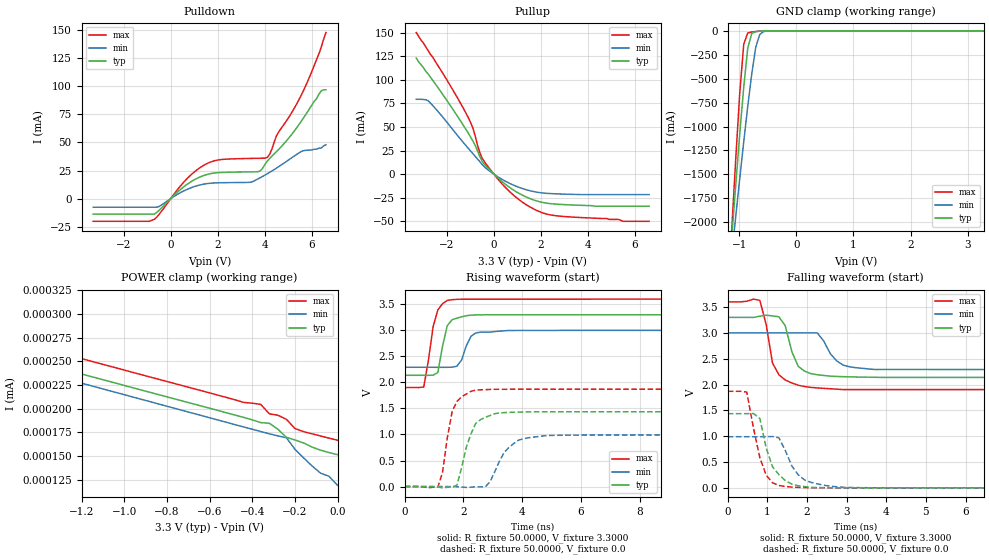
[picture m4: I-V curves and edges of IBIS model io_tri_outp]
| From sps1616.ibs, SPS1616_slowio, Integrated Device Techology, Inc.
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|   Model io_tri_outp
[Model]  io_tri_outp
Model_type 3-state
Polarity   Non-Inverting
Enable   Active-Low
Vmeas =  1.6500V
Cref =   50.0000pF
Rref =   1.0000M
Vref =   0.0V
C_comp   2.4707pF   2.4446pF   2.5092pF
[Temperature Range]   25.0000   0.1250k   -40.0000
[Voltage Range]   3.3000V   3.0000V   3.6000V
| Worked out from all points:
|   slope of the pulldown table from 0 to 0.495 V, typ, clamps not added: 51.9 ohm
|   slope of the pullup table from 0 to 0.495 V, typ, clamps not added: 45.6 ohm
|   GND clamp passes 1 mA (typ) near -0.54 V on its own axis
|   POWER clamp passes 1 mA (typ) near -2.49 V on its own axis
|   rising waveform, R_fixture 50.0000, V_fixture 3.3000: 20-80 % time 254ps typ, 295ps min, 311ps max; typ from 2.14 V to 3.3 V
|   rising waveform, R_fixture 50.0000, V_fixture 0.0: 20-80 % time 465ps typ, 642ps min, 346ps max; typ from 0 V to 1.44 V
|   falling waveform, R_fixture 50.0000, V_fixture 3.3000: 20-80 % time 295ps typ, 393ps min, 317ps max; typ from 3.3 V to 2.14 V
|   falling waveform, R_fixture 50.0000, V_fixture 0.0: 20-80 % time 393ps typ, 459ps min, 342ps max; typ from 1.44 V to 0 V
[Pulldown]
|Voltage   I(typ)   I(min)   I(max)
-3.3V     -13.86mA   -7.71mA    -20.27mA
-900mV    -13.86mA   -7.71mA    -20.27mA
-600mV    -12.36mA   -7.71mA    -16.59mA
700mV     12.78mA    8.245mA    17.92mA
1.5V      21.21mA    13.2mA     30.77mA
2.1V      23.2mA     14.09mA    34.69mA
3.7V      23.92mA    17.44mA    35.89mA
4.1V      33.25mA    22.07mA    36.63mA
4.5V      41.93mA    27.2mA     56.15mA
5.7V      73.6mA     42.86mA    98.81mA
6.4V      96mA       45mA       135mA
6.6V      97mA       48mA       148mA
[Pullup]
|Voltage   I(typ)   I(min)   I(max)
-3.3V     123mA      79.3mA     150mA
-2.8V     106.3mA    77.79mA    131mA
-1.2V     47.86mA    30.59mA    65.19mA
-900mV    35.42mA    21.89mA    49.37mA
-600mV    18.69mA    13.25mA    22.89mA
-500mV    13.73mA    10.33mA    16.95mA
300mV     -6.88mA    -4.819mA   -8.986mA
1V        -19.4mA    -13.37mA   -25.69mA
1.7V      -27.44mA   -18.53mA   -37.02mA
2.4V      -31.25mA   -20.6mA    -43.2mA
5.5V      -34mA      -21.7mA    -50mA
6.6V      -34mA      -21.7mA    -50mA
[GND_clamp]
|Voltage   I(typ)   I(min)   I(max)
-3.3V     -20.24A    -15.41A    -26.98A
-1.13V    -2.159A    -2.344A    -2.077A
-1.06V    -1.611A    -1.941A    -1.338A
-990mV    -1.08A     -1.545A    -651.6mA
-920mV    -586.7mA   -1.158A    -139.4mA
-850mV    -181.3mA   -789.1mA   -22.48mA
-780mV    -28.37mA   -450.9mA   -12.35mA
-710mV    -7.599mA   -171.5mA   -7.64mA
-640mV    -3.504mA   -37.73mA   -3.899mA
-570mV    -1.414mA   -7.386mA   -1.365mA
-360mV    -3.781uA   -39.23uA   -907.8nA
3.28V     150.3nA    317.1nA    148.8nA
[POWER_clamp]
|Voltage   I(typ)   I(min)   I(max)
-3.28V    3.127A     1.353A     6.658A
-2.28V    531.3nA    314.4nA    683.5uA
-2.24V    350.6nA    298.4nA    96.38uA
-2.12V    294.9nA    284.6nA    571.2nA
-2.04V    289.2nA    279.3nA    310.9nA
-1.96V    283.9nA    274.2nA    300.7nA
-1.44V    251.4nA    241.7nA    267.6nA
-360mV    185.4nA    176nA      204.6nA
-320mV    184.7nA    173.6nA    194.7nA
-240mV    169.9nA    169.4nA    188.9nA
-200mV    167.1nA    157.3nA    179.2nA
0V        151.5nA    119.1nA    166.8nA
[Ramp]
| variable   typ   min   max
dV/dt_r  0.8616/0.4648n   0.5939/0.6317n   1.1214/0.3356n
dV/dt_f  0.6978/0.2866n   0.4254/0.3829n   1.0188/0.3174n
R_load = 50.0000
[Rising Waveform]
R_fixture= 50.0000
V_fixture= 3.3000
V_fixture_min= 3.0000
V_fixture_max= 3.6000
L_fixture= 0.0H
C_fixture= 0.0F
|time   V(typ)   V(min)   V(max)
0s        2.137V     2.291V     1.902V
650ps     2.137V     2.291V     1.912V
970ps     2.139V     2.291V     3.074V
1.13ns    2.19V      2.29V      3.393V
1.45ns    3.089V     2.29V      3.575V
1.78ns    3.234V     2.312V     3.596V
1.94ns    3.26V      2.431V     3.598V
2.26ns    3.293V     2.886V     3.599V
2.59ns    3.297V     2.967V     3.599V
16ns      3.3V       3V         3.6V
[Rising Waveform]
R_fixture=   50.0000
V_fixture=   0.0
V_fixture_min= 0.0
V_fixture_max= 0.0
L_fixture=   0.0H
C_fixture=   0.0F
|time   V(typ)   V(min)   V(max)
0s        2.775uV    3.203uV    2.534uV
1.13ns    -8.238mV   55.76uV    -11.81mV
1.29ns    -25.11mV   29.81uV    268.3mV
1.62ns    -9.698mV   -1.144mV   1.447V
1.78ns    25.31mV    -3.255mV   1.634V
2.42ns    1.213V     -5.268mV   1.853V
2.75ns    1.33V      -4.111mV   1.861V
3.39ns    1.42V      654.6mV    1.868V
4.2ns     1.434V     935.4mV    1.87V
16ns      1.436V     989.8mV    1.869V
[Falling Waveform]
R_fixture=   50.0000
V_fixture=   3.3000
V_fixture_min= 3.0000
V_fixture_max= 3.6000
L_fixture=   0.0H
C_fixture=   0.0F
|time   V(typ)   V(min)   V(max)
0s        3.3V       3V         3.6V
810ps     3.323V     3V         3.629V
1.13ns    3.328V     3V         2.414V
1.29ns    3.311V     3V         2.19V
1.45ns    3.14V      3V         2.088V
1.78ns    2.351V     3V         1.986V
2.1ns     2.21V      3V         1.944V
2.91ns    2.152V     2.376V     1.902V
3.72ns    2.14V      2.291V     1.902V
16ns      2.137V     2.291V     1.902V
[Falling Waveform]
R_fixture= 50.0000
V_fixture= 0.0
V_fixture_min= 0.0
V_fixture_max= 0.0
L_fixture= 0.0H
C_fixture= 0.0F
|time   V(typ)   V(min)   V(max)
0s        1.436V     989.8mV    1.869V
480ps     1.436V     989.8mV    1.853V
810ps     1.343V     989.7mV    585.8mV
1.13ns    407.2mV    992.8mV    97.92mV
1.29ns    257mV      969.6mV    45.92mV
1.45ns    142.7mV    726.6mV    27.17mV
1.62ns    71.16mV    419.2mV    14.69mV
1.94ns    24.65mV    152.4mV    5.349mV
2.91ns    1.536mV    11.88mV    336.6uV
16ns      18.3uV     0V         -10.41uV
